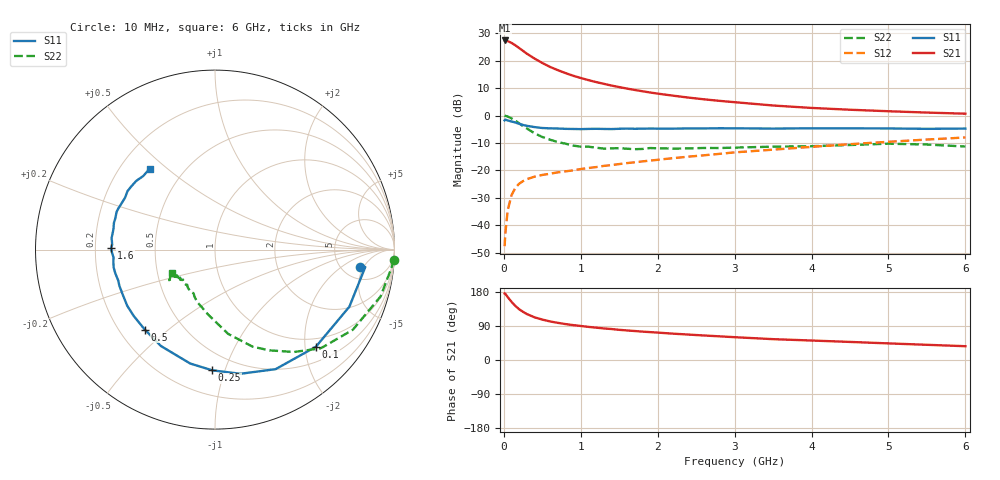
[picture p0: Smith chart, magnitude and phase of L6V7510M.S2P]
!  INFINEON TECHNOLOGIES Small Signal Semiconductors
! BFR380L3 , Si-NPN RF-Transistor in TSLP-3-1
!  Vce=0.75 V,  Ic=10 mA
! Common Emitter S-Parameters:  07. March 2005
#  GHz  S  MA  R  50
! f  S11  S21  S12  S22
! GHz  Mag  Ang  Mag  Ang  Mag  Ang  Mag  Ang
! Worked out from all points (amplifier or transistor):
!   36 points, 10 MHz to 6 GHz, reference 50 ohm
!   highest |S21| = 27.3 dB at 10 MHz (marker M1)
!   |S21| within 3 dB of that: start of sweep to 210.6 MHz
!   unconditionally stable (mu >= 1): 1.968 GHz to 5.428 GHz
!   at 250 MHz: K = 0.27, MSG = 23.7 dB, |S12| = -23.9 dB
!   at 1.4 GHz: K = 0.91, MSG = 14.5 dB, |S12| = -18.0 dB
!   at 6 GHz: K = 0.99, MSG = 4.3 dB, |S12| = -8.0 dB
!   S11 on the Smith chart (normalised r, x): 10 MHz: 7.26, -4.33; 100 MHz: 0.81, -2.23; 250 MHz: 0.37, -0.91; 500 MHz: 0.30, -0.42; 1.6 GHz: 0.27, +0.01; 6 GHz: 0.32, +0.44
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0.01  0.8162 -7.0  23.22 175.5  0.0042 85.5  0.9999 -3.2
0.02  0.8429 -6.6  23.02 174.6  0.0073 85.8  0.9858 -6.5
0.05  0.8135 -23.0  22.59 166.0  0.0189 79.7  0.9587 -15.8
0.1  0.7803 -43.9  20.95 153.5  0.0356 69.6  0.8883 -30.2
0.15  0.7468 -63.1  18.95 142.6  0.0484 61.0  0.8058 -43.1
0.2  0.7063 -78.4  16.85 133.8  0.0576 56.0  0.72 -52.4
0.25  0.6728 -91.3  15.01 127.1  0.0641 50.9  0.6382 -61.6
0.3  0.6495 -102.3  13.33 121.2  0.0696 48.2  0.5803 -68.8
0.4  0.6159 -119.3  10.85 112.6  0.0773 44.6  0.4756 -81.1
0.5  0.5928 -131.3  9.043 106.6  0.083 43.4  0.407 -88.8
0.6  0.5847 -140.7  7.674 101.8  0.0874 42.9  0.3631 -96.2
0.7  0.5806 -147.4  6.702 98.1  0.0925 44.1  0.3294 -102.9
0.9  0.5697 -159.2  5.299 92.1  0.1005 45.4  0.284 -113.9
1.1  0.5708 -166.5  4.406 87.4  0.1109 47.5  0.271 -120.6
1.4  0.567 -175.5  3.509 81.7  0.1255 50.1  0.253 -128.6
1.6  0.579 179.1  3.094 78.0  0.1363 51.4  0.249 -136.0
2.2  0.5776 168.2  2.298 69.5  0.1677 54.8  0.2502 -140.3
2.8  0.5873 159.0  1.851 62.5  0.2005 57.1  0.2564 -146.1
3.5  0.5785 150.1  1.522 55.0  0.2395 56.9  0.2715 -146.2
4.5  0.5845 143.2  1.275 47.7  0.3009 57.0  0.2907 -146.5
5.5  0.5726 134.3  1.132 40.1  0.3655 54.3  0.2968 -147.7
6  0.5793 128.9  1.08 36.4  0.3991 52.6  0.2728 -151.4
